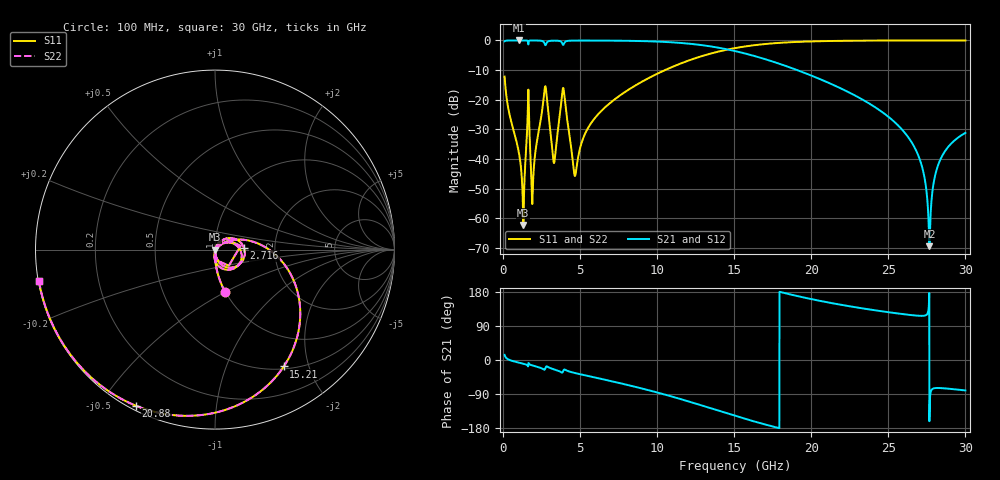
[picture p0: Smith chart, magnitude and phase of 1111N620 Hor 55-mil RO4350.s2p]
# GHz S MA R 50
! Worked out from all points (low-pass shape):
!   3201 points, 100 MHz to 30 GHz, reference 50 ohm
!   highest |S21| = -0.01 dB at 1.025 GHz (marker M1); lowest = -69.3 dB at 27.66 GHz (marker M2)
!   |S21| within 3 dB of the highest: start of sweep to 14.54 GHz
!   lowest |S11| = -62.2 dB at 1.315 GHz (marker M3), VSWR 1.00, Z = 50.1 - j0.0259 ohm
!   |S11| at or under -10 dB: start of sweep to 10.51 GHz
!   |S22| runs from -62.2 to 0.0 dB; largest |S21 - S12| = 0
!   S11 on the Smith chart (normalised r, x): 100 MHz: 0.99, -0.50; 2.716 GHz: 1.39, +0.03; 15.21 GHz: 0.53, -1.62; 20.88 GHz: 0.02, -0.61; 30 GHz: 0.00, -0.09
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0.1  0.2453 -76.5  0.9692 13.4  0.9692 13.4  0.2453 -76.5
1.025031  0.01288 -94.7  0.9993 -7.0  0.9993 -7.0  0.01288 -94.7
1.314688  0.0007764 -19.5  0.9991 -9.9  0.9991 -9.9  0.0007764 -19.5
1.595  0.05416 57.6  0.9822 -14.9  0.9822 -14.9  0.05416 57.6
1.950063  0.00436 52.7  0.9981 -14.8  0.9981 -14.8  0.00436 52.7
2.71625  0.1628 3.2  0.8527 -24.6  0.8527 -24.6  0.1628 3.2
3.286219  0.008755 -30.7  0.9909 -24.4  0.9909 -24.4  0.008755 -30.7
3.893562  0.1582 -23.3  0.8422 -29.9  0.8422 -29.9  0.1582 -23.3
4.622375  0.005586 -47.7  0.994 -34.0  0.994 -34.0  0.005586 -47.7
5.089563  0.01863 40.4  0.9956 -38.4  0.9956 -38.4  0.01863 40.4
6.621937  0.07465 35.8  0.9938 -52.2  0.9938 -52.2  0.07465 35.8
10.06978  0.2798 2.9  0.9557 -86.5  0.9557 -86.5  0.2798 2.9
15.05  0.743 -57.6  0.6621 -147.2  0.6621 -147.2  0.743 -57.6
15.20884  0.7556 -59.5  0.6477 -149.1  0.6477 -149.1  0.7556 -59.5
20.03956  0.9636 -110.0  0.2536 160.4  0.2536 160.4  0.9636 -110.0
20.8805  0.9752 -116.8  0.2057 153.5  0.2057 153.5  0.9752 -116.8
25.01978  0.9957 -144.7  0.0513 126.0  0.0513 126.0  0.9957 -144.7
26.92591  0.997 -155.1  0.01181 116.9  0.01181 116.9  0.997 -155.1
27.32769  0.997 -157.2  0.005188 116.9  0.005188 116.9  0.997 -157.2
27.66406  0.997 -158.9  0.0003411 -161.6  0.0003411 -161.6  0.997 -158.9
28.34616  0.997 -162.2  0.009455 -74.0  0.009455 -74.0  0.997 -162.2
30  0.9966 -169.9  0.02766 -80.3  0.02766 -80.3  0.9966 -169.9
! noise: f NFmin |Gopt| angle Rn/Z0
0.1  0.0006342  0.7235  1.521  0.000455
3.417  0.02289  0.7397  25.35  0.01679
6.743  0.01866  0.4832  47.43  0.005289
10.06  0.02541  0.469  65.04  0.00606
13.39  0.03707  0.5353  80.72  0.00873
16.7  0.05881  0.6549  97.58  0.01489
20.03  0.108  0.7931  116.7  0.03075
23.35  0.2569  0.9077  136  0.08711
26.67  1.551  0.9838  153.9  1.136
30  0.9361  0.9725  169.8  0.06264
